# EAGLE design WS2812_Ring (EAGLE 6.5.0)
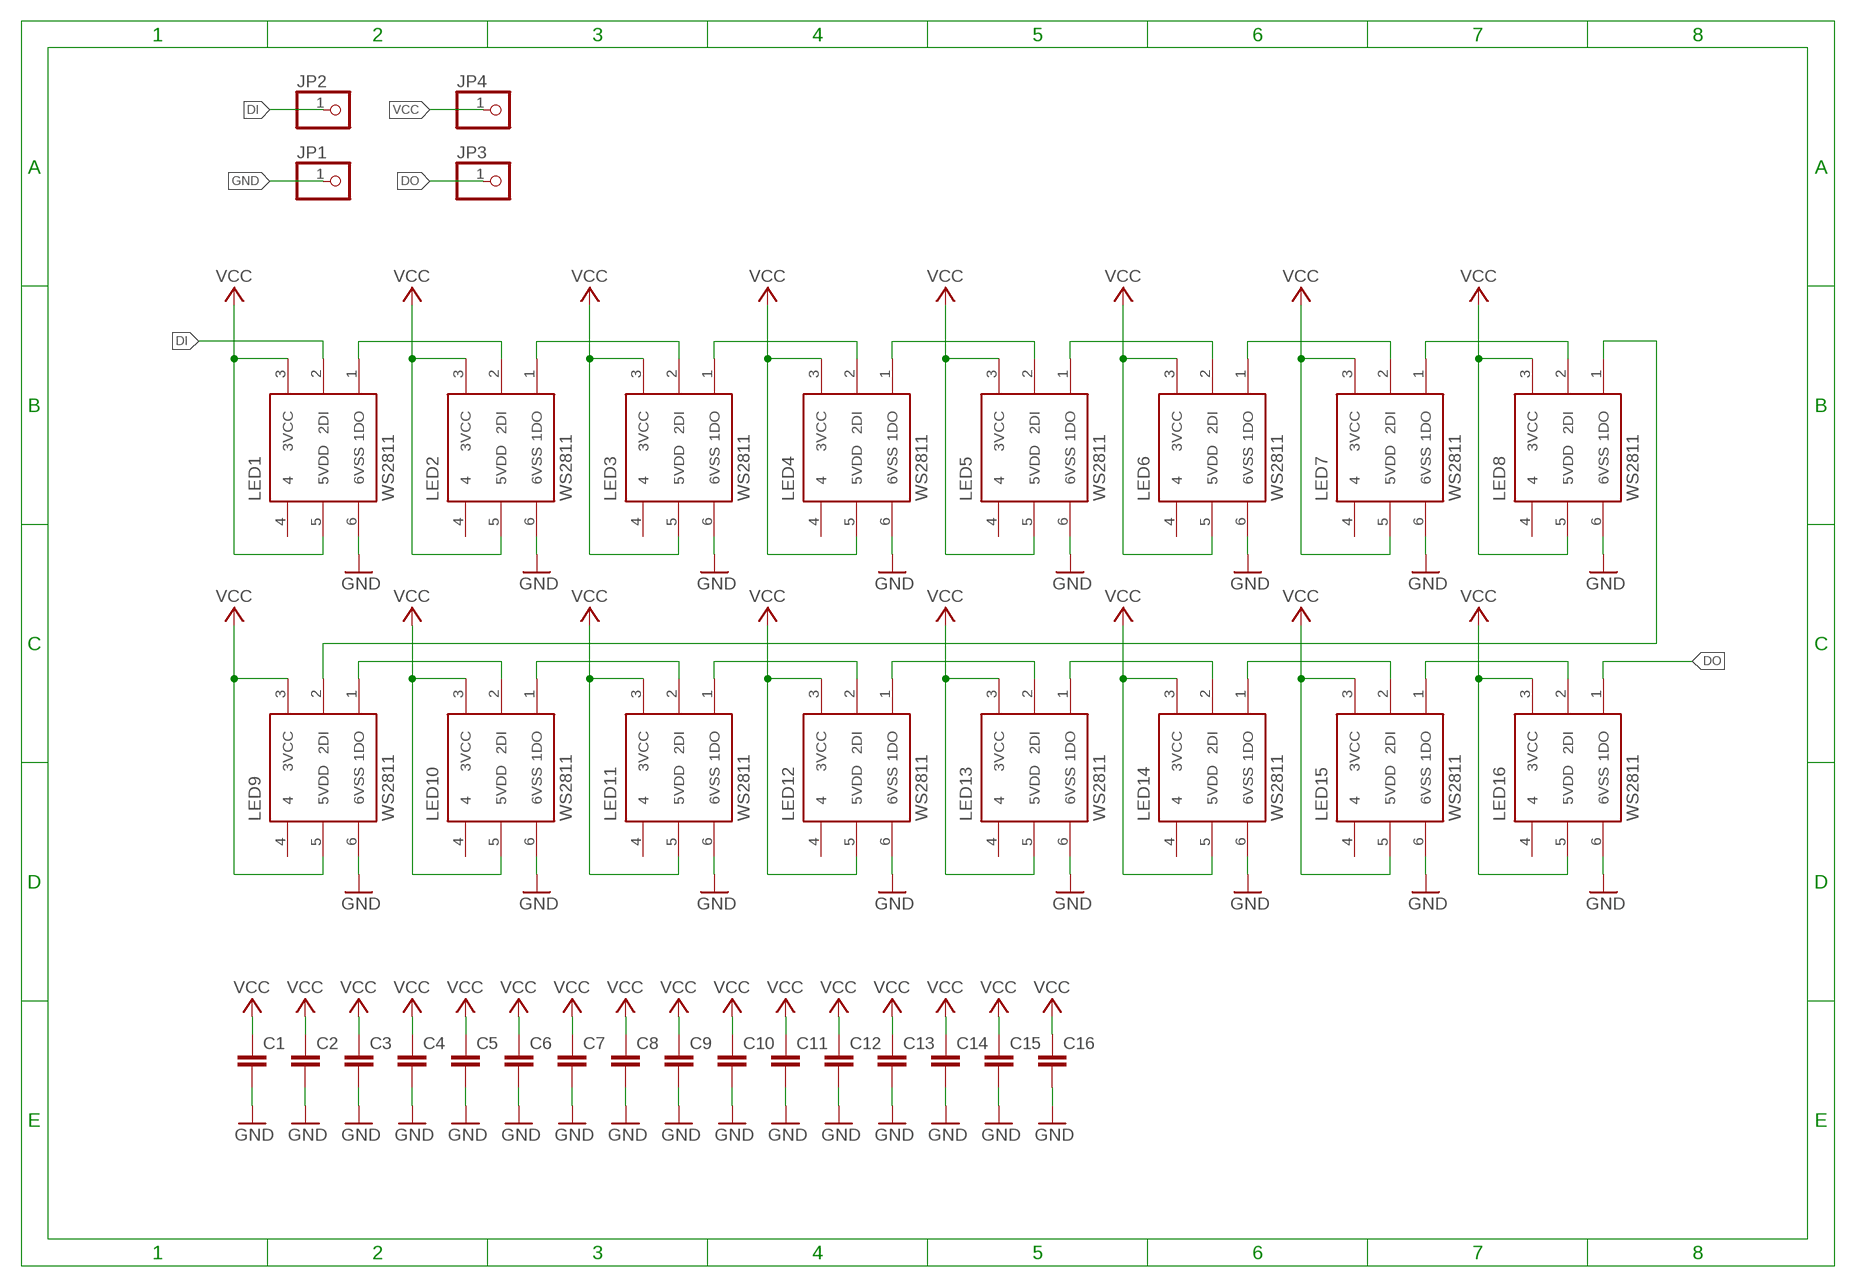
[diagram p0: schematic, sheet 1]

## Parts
C1  C-EUC0805  [C0805]
C2  C-EUC0805  [C0805]
C3  C-EUC0805  [C0805]
C4  C-EUC0805  [C0805]
C5  C-EUC0805  [C0805]
C6  C-EUC0805  [C0805]
C7  C-EUC0805  [C0805]
C8  C-EUC0805  [C0805]
C9  C-EUC0805  [C0805]
C10  C-EUC0805  [C0805]
C11  C-EUC0805  [C0805]
C12  C-EUC0805  [C0805]
C13  C-EUC0805  [C0805]
C14  C-EUC0805  [C0805]
C15  C-EUC0805  [C0805]
C16  C-EUC0805  [C0805]
JP1  PINHD-1X1  [1X01]
JP2  PINHD-1X1  [1X01]
JP3  PINHD-1X1  [1X01]
JP4  PINHD-1X1  [1X01]
LED1  WS2811  [WS2812]
LED2  WS2811  [WS2812]
LED3  WS2811  [WS2812]
LED4  WS2811  [WS2812]
LED5  WS2811  [WS2812]
LED6  WS2811  [WS2812]
LED7  WS2811  [WS2812]
LED8  WS2811  [WS2812]
LED9  WS2811  [WS2812]
LED10  WS2811  [WS2812]
LED11  WS2811  [WS2812]
LED12  WS2811  [WS2812]
LED13  WS2811  [WS2812]
LED14  WS2811  [WS2812]
LED15  WS2811  [WS2812]
LED16  WS2811  [WS2812]

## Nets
DI: JP2.1 LED1.2(2DI)
DO: JP3.1 LED16.1(1DO)
GND: C1.2 C2.2 C3.2 C4.2 C5.2 C6.2 C7.2 C8.2 C9.2 C10.2 C11.2 C12.2 C13.2 C14.2 C15.2 C16.2 JP1.1 LED1.6(6VSS) LED2.6(6VSS) LED3.6(6VSS) LED4.6(6VSS) LED5.6(6VSS) LED6.6(6VSS) LED7.6(6VSS) LED8.6(6VSS) LED9.6(6VSS) LED10.6(6VSS) LED11.6(6VSS) LED12.6(6VSS) LED13.6(6VSS) LED14.6(6VSS) LED15.6(6VSS) LED16.6(6VSS)
N$2: LED1.1(1DO) LED2.2(2DI)
N$3: LED2.1(1DO) LED3.2(2DI)
N$4: LED3.1(1DO) LED4.2(2DI)
N$5: LED4.1(1DO) LED5.2(2DI)
N$6: LED5.1(1DO) LED6.2(2DI)
N$7: LED7.1(1DO) LED8.2(2DI)
N$8: LED9.1(1DO) LED10.2(2DI)
N$9: LED10.1(1DO) LED11.2(2DI)
N$10: LED11.1(1DO) LED12.2(2DI)
N$11: LED12.1(1DO) LED13.2(2DI)
N$12: LED13.1(1DO) LED14.2(2DI)
N$13: LED15.1(1DO) LED16.2(2DI)
N$14: LED8.1(1DO) LED9.2(2DI)
N$15: LED6.1(1DO) LED7.2(2DI)
N$17: LED14.1(1DO) LED15.2(2DI)
VCC: C1.1 C2.1 C3.1 C4.1 C5.1 C6.1 C7.1 C8.1 C9.1 C10.1 C11.1 C12.1 C13.1 C14.1 C15.1 C16.1 JP4.1 LED1.3(3VCC) LED1.5(5VDD) LED2.3(3VCC) LED2.5(5VDD) LED3.3(3VCC) LED3.5(5VDD) LED4.3(3VCC) LED4.5(5VDD) LED5.3(3VCC) LED5.5(5VDD) LED6.3(3VCC) LED6.5(5VDD) LED7.3(3VCC) LED7.5(5VDD) LED8.3(3VCC) LED8.5(5VDD) LED9.3(3VCC) LED9.5(5VDD) LED10.3(3VCC) LED10.5(5VDD) LED11.3(3VCC) LED11.5(5VDD) LED12.3(3VCC) LED12.5(5VDD) LED13.3(3VCC) LED13.5(5VDD) LED14.3(3VCC) LED14.5(5VDD) LED15.3(3VCC) LED15.5(5VDD) LED16.3(3VCC) LED16.5(5VDD)
Unconnected: LED1.4 LED2.4 LED3.4 LED4.4 LED5.4 LED6.4 LED7.4 LED8.4 LED9.4 LED10.4 LED11.4 LED12.4 LED13.4 LED14.4 LED15.4 LED16.4

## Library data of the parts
C1-C16 = rcl:C-EU: CAPACITOR, European symbol
JP1-JP4 = pinhead:PINHD-1X1: PIN HEADER
LED1-LED16 = led2:WS2811

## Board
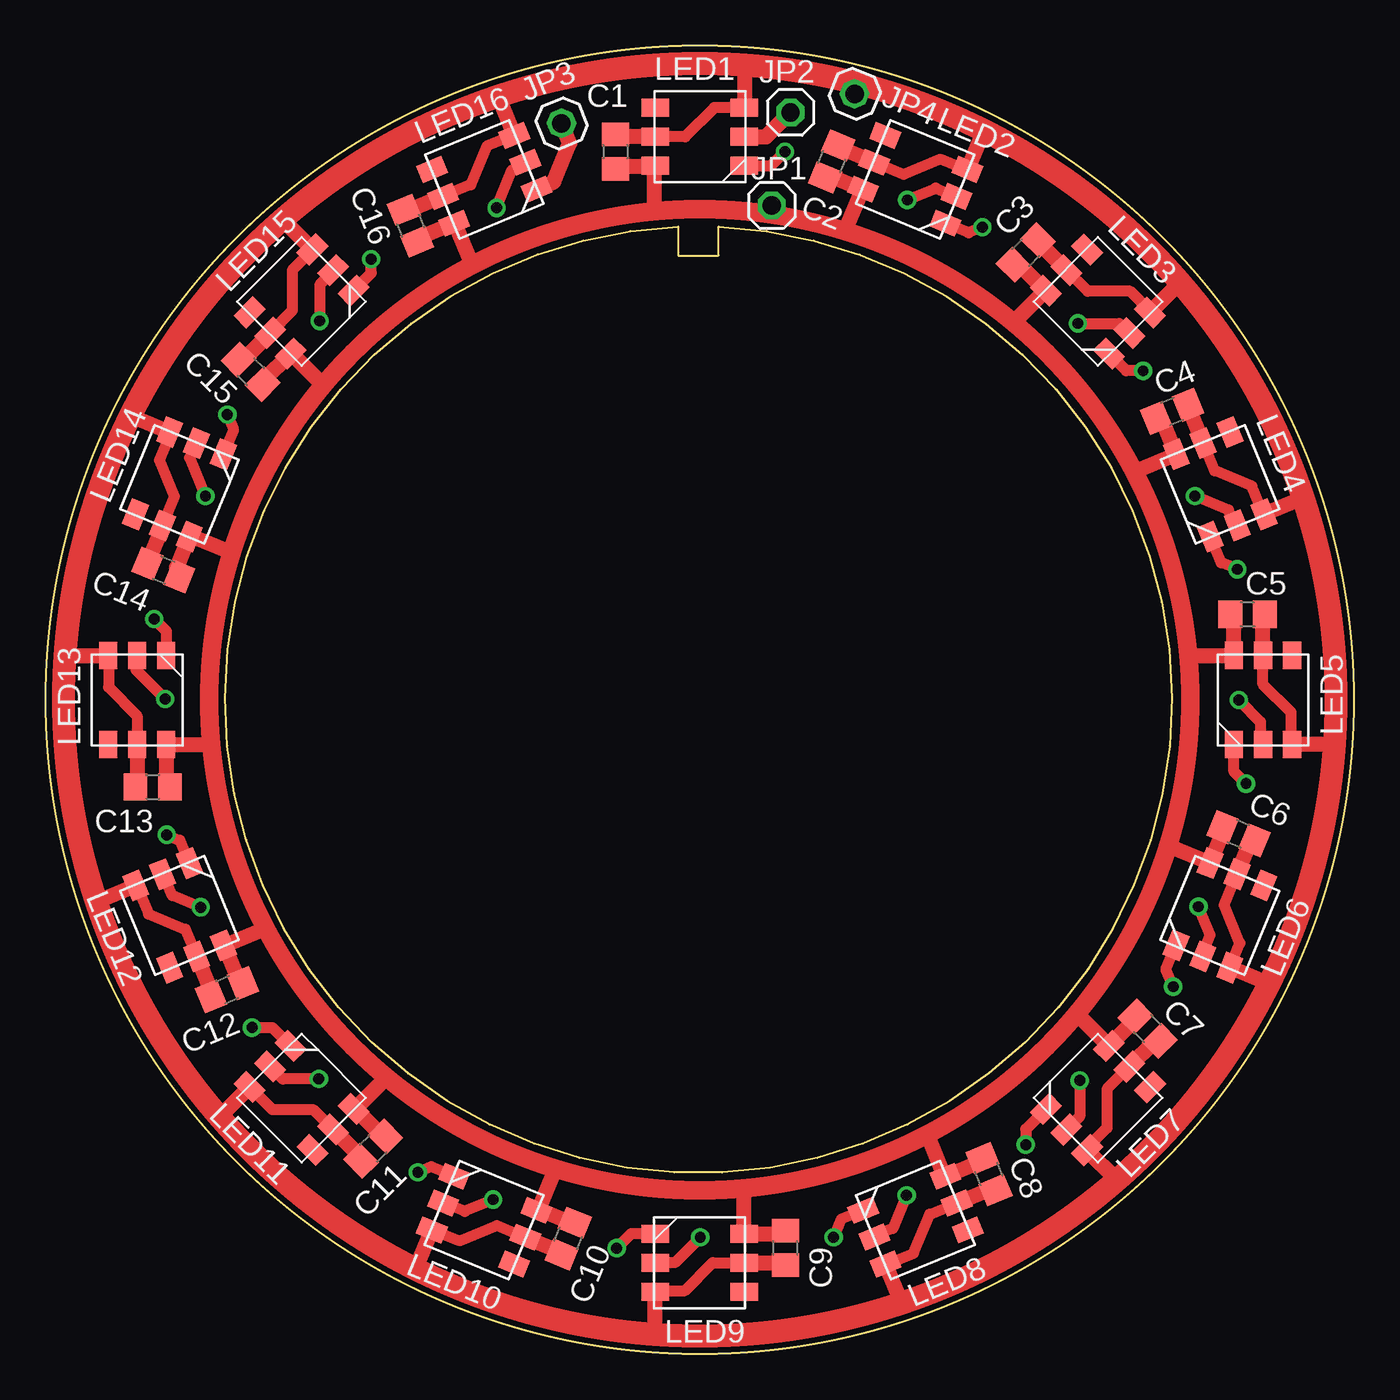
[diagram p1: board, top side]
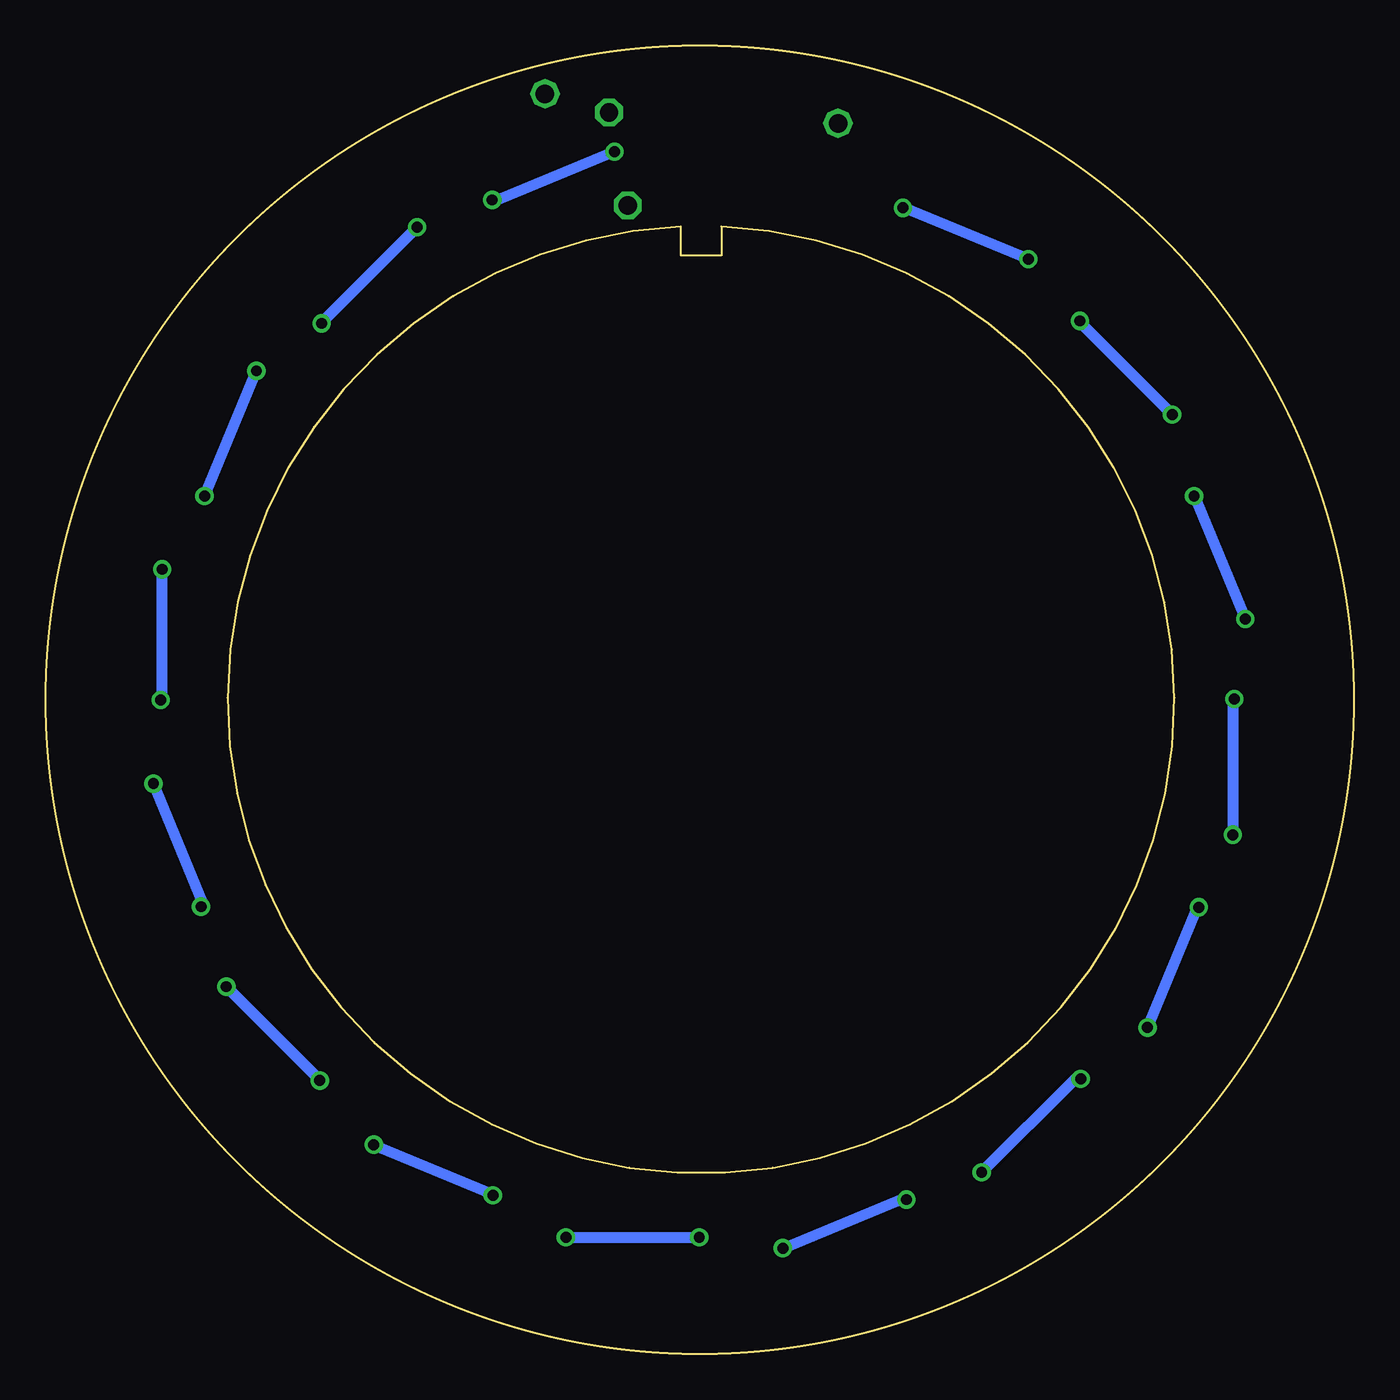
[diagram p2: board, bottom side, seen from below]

Size 72.03 x 72.03 mm. Coordinates in mm from the lower left corner, seen from the top.
Outline: 34.83,62.05 34.83,60.46 37.05,60.46 37.05,62.05 arc-355 34.83,62.05
Outline: circle at 36.01,36.01 radius 36.01
Copper layers (1*16): Top 0.035mm / dielectric 1.5mm / Bottom 0.035mm
Design rules "default": minimum track width 10mil, minimum drill 24mil, track to track 8mil, track to pad 8mil, pad to pad 8mil, via to via 8mil, smd to smd 8mil, copper to edge 40mil, drill to drill 8mil, minimum pad ring 10mil, minimum via ring 8mil, stop-mask expansion 4mil, vias tented up to drill 0mil, thermal gap 10mil

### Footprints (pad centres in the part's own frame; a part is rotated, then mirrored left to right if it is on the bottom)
C0805 = smd 1.3 x 1.5: 1 -0.95,0; 2 0.95,0
1X01 = drill 1.016 octagon: 1 0,0
WS2812 = smd 1.5 x 1: 1 2.45,-1.6; 2 2.45,0; 3 2.45,1.6; 4 -2.45,1.6; 5 -2.45,0; 6 -2.45,-1.6

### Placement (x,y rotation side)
C1  31.37,66.18 270 top
C2  43.28,65.65 247.5 top
C3  53.95,60.63 225 top
C4  62.01,51.88 202.5 top
C5  66.16,40.71 180 top
C6  65.67,28.64 157.5 top
C7  60.66,17.91 135 top
C8  51.93,9.91 112.5 top
C9  40.73,5.85 90 top
C10  28.77,6.35 67.5 top
C11  18.04,11.31 45 top
C12  9.99,20.06 22.5 top
C13  5.9,31.22 0 top
C14  6.49,43.15 337.5 top
C15  11.29,54.07 315 top
C16  20.09,62.1 292.5 top
JP1  39.97,63.22 0 top
JP2  41.01,68.35 0 top
JP3  28.4,67.74 22.5 top
JP4  44.53,69.36 337.5 top
LED1  36.02,67 0 top
LED2  47.88,64.66 337.5 top
LED3  57.93,57.93 315 top
LED4  64.66,47.87 292.5 top
LED5  67.01,36.01 270 top
LED6  64.64,24.15 247.5 top
LED7  57.93,14.09 225 top
LED8  47.89,7.37 202.5 top
LED9  36.01,5.03 180 top
LED10  24.15,7.37 157.5 top
LED11  14.1,14.1 135 top
LED12  7.38,24.14 112.5 top
LED13  5.05,36 90 top
LED14  7.38,47.87 67.5 top
LED15  14.09,57.94 45 top
LED16  24.15,64.66 22.5 top

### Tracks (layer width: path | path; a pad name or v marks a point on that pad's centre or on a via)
DI
  Top 0.813: LED1.2 39.66,67 JP2.1
DO
  Top 0.813: LED16.1 27.98,64.51 28.86,66.63 JP3.1
GND
  Top 0.305: 33.52,65.35 LED1.6 | 61.81,28.01 62.31,30.11 arc17 62.91,34.11 62.91,38.46 62.91,38.51 62.41,41.81 61.41,45.11 60.01,48.61 59.41,49.31 58.01,51.61 55.71,54.51 53.31,56.81 52.61,57.31 51.41,58.11 49.11,59.61 46.61,60.81 44.01,61.81 42.31,62.21 40.01,62.61 37.11,62.91 33.52,62.91 31.02,62.51 | 61.81,28.01 60.81,25.22 59.11,22.02 56.82,18.77 | 56.82,18.77 56.71,18.62 55.01,16.82 52.71,14.82 50.21,13.02 48.51,12.12 45.61,10.72 41.81,9.62 38.41,9.12 34.82,9.02 31.72,9.32 29.32,9.82 28.06,10.18 27.92,10.22 26.02,10.92 23.42,12.02 21.62,13.12 19.72,14.42 18.62,15.32 | 18.62,15.32 17.02,16.82 14.82,19.22 13.52,21.11 12.12,23.51 | 31.02,62.51 28.12,61.81 25.62,60.91 23.52,59.91 | 15.32,53.31 14.92,52.61 13.52,50.91 11.32,46.71 10.22,44.11 9.63,41.85 9.19,39.22 9.04,36.25 9.02,34.1 9.12,33.51 arc7 9.62,30.01 arc15 11.32,25.11 12.12,23.51 | 6.69,33.51 LED13.6 | 61.81,28.01 61.83,27.96 | 56.82,18.67 56.82,18.77 | 49.46,9.82 LED8.6 | 38.41,6.67 LED9.6 | 27.15,7.96 LED10.6 | 17.04,13.5 LED11.6 | 18.62,15.32 18.74,15.2 | 9.84,22.48 LED12.6 | 12.12,23.51 12.15,23.43 | 8,45.03 LED14.6 | 13.56,55.07 LED15.6 | 22.56,62.22 LED16.6 | 44.96,64.1 LED2.6 | 55.03,58.53 LED3.6 | 62.23,49.53 LED4.6 | 65.41,40.51 C5.2 | 64.86,28.85 C6.2 | 59.99,18.41 arc180 C7.2 | 51.49,10.6 arc180 C8.2 | 40.56,6.63 arc180 C9.2 | 29.03,7.18 arc180 C10.2 | 18.55,11.98 C11.2 | 10.65,20.51 C12.2 | 6.65,31.42 C13.2 | 7.21,43.3 7.2,43.29 7.18,43.25 C14.2 | 11.97,53.54 C15.2 | 20.54,61.43 C16.2 | 31.49,65.35 C1.2 | 43.13,64.86 C2.2 | 53.61,59.95 C3.2 | 61.47,51.38 C4.2 | 31.02,62.51 30.67,62.36 JP1.1
  Top 0.813: 33.52,62.91 33.52,65.35 31.49,65.35 | 62.91,38.46 LED5.6 65.41,40.51 | 61.83,27.96 LED6.6 64.86,28.85 | 56.82,18.67 LED7.6 59.99,18.41 | 48.51,12.12 49.46,9.82 | 38.41,9.12 38.41,6.67 | 28.06,10.18 27.15,7.96 29.03,7.18 | 18.74,15.2 17.04,13.5 18.55,11.98 | 12.15,23.43 9.84,22.48 10.65,20.51 | 9.12,33.51 6.69,33.51 | 10.22,44.11 8,45.03 | 15.32,53.31 13.56,55.07 | 23.52,59.91 22.56,62.22 | 44.01,61.81 44.96,64.1 43.13,64.86 | 53.31,56.81 55.03,58.53 53.61,59.95 | 60.01,48.61 62.23,49.53 61.47,51.38 | LED8.6 51.49,10.6 | LED9.6 40.56,6.63 | LED13.6 6.65,31.42 | LED14.6 7.21,43.3 | LED15.6 11.97,53.54 | LED16.6 20.54,61.43
N$2  (via drill 0.6)
  Top 0.305: 50.12,63.71 LED2.2
  Top 0.61: LED1.1 39.93,65.4 v40.71,66.18 | v47.43,63.53 49,64.17 50.12,63.71
  Bottom 0.305: 47.27,63.46 v47.43,63.53
  Bottom 0.61: v40.71,66.18 47.27,63.46
N$3  (via drill 0.6)
  Top 0.305: 59.62,56.2 LED3.2
  Top 0.61: LED2.1 50.81,61.71 v51.58,62.03 | v56.83,56.73 59.09,56.73 59.62,56.2
  Bottom 0.305: 56.83,56.77 v56.83,56.73
  Bottom 0.61: v51.58,62.03 56.83,56.77
N$4  (via drill 0.6)
  Top 0.305: LED4.2 65.44,45.67 | 65.12,46.46 65.54,45.43 65.56,45.42
  Top 0.61: 65.44,45.67 65.12,46.46 v63.27,47.22 | LED3.1 59.48,54.12 v60.41,54.12
  Bottom 0.61: v63.27,47.22 v60.41,54.12
N$5  (via drill 0.6)
  Top 0.305: 66.88,33.69 LED5.2
  Top 0.61: LED4.1 64.71,43.56 v65.6,43.2 | v65.68,36 66.88,34.8 66.88,33.69
  Bottom 0.305: v65.68,36 65.6,36.07
  Bottom 0.61: 65.6,36.07 v65.6,43.2
N$6  (via drill 0.6)
  Top 0.305: LED6.2 63.67,21.98
  Top 0.61: LED5.1 65.41,32.06 v66.08,31.4 | v63.46,24.62 64.11,23.06 63.67,21.98
  Bottom 0.305: v63.46,24.62 63.37,24.85
  Bottom 0.61: 63.37,24.85 v66.08,31.4
N$7  (via drill 0.6)
  Top 0.305: 45.65,6.5 LED8.2
  Top 0.61: LED7.1 53.96,12.38 v53.96,11.52 | v47.4,8.74 46.64,6.91 45.65,6.5
  Bottom 0.305: 47.43,8.82 v47.4,8.74
  Bottom 0.61: v53.96,11.52 47.43,8.82
N$8  (via drill 0.6)
  Top 0.305: 21.93,8.33 LED10.2
  Top 0.61: LED9.1 32.24,6.63 v31.44,5.83 | v24.64,8.5 23.07,7.85 21.93,8.33
  Bottom 0.305: 24.81,8.58 v24.64,8.5
  Bottom 0.61: v31.44,5.83 24.81,8.58
N$9  (via drill 0.6)
  Top 0.305: 12.39,15.83 LED11.2
  Top 0.61: LED10.1 21.24,10.31 v20.5,10 | v15.05,15.15 13.07,15.15 12.39,15.83
  Bottom 0.305: 15.35,15.15 v15.05,15.15
  Bottom 0.61: v20.5,10 15.35,15.15
N$10  (via drill 0.6)
  Top 0.305: 6.51,26.38 LED12.2
  Top 0.61: LED11.1 12.48,17.97 v11.37,17.97 | v8.55,24.59 6.98,25.24 6.51,26.38
  Bottom 0.305: v8.55,24.59 8.65,24.55
  Bottom 0.61: 8.65,24.55 v11.37,17.97
N$11  (via drill 0.6)
  Top 0.305: 4.99,37.65 4.99,38.38 LED13.2
  Top 0.61: LED12.1 7.4,28.28 v6.68,28.58 | 4.99,37.65 v6.59,36.05
  Bottom 0.305: v6.59,36.05 6.68,35.96
  Bottom 0.61: 6.68,35.96 v6.68,28.58
N$12  (via drill 0.6)
  Top 0.305: LED14.2 8.27,50.12
  Top 0.61: LED13.1 6.65,39.79 v5.99,40.45 | v8.81,47.23 7.94,49.32 8.27,50.12
  Bottom 0.305: v8.81,47.23 8.79,47.22
  Bottom 0.61: 8.79,47.22 v5.99,40.45
N$13  (via drill 0.6)
  Top 0.305: 26.36,65.46 LED16.2
  Top 0.61: LED15.1 17.93,59.5 v17.93,60.26 | v24.83,63.09 25.69,65.18 26.36,65.46
  Bottom 0.305: 24.79,63.11 v24.83,63.09
  Bottom 0.61: v17.93,60.26 24.79,63.11
N$14  (via drill 0.6)
  Top 0.305: LED9.2
  Top 0.61: LED8.1 43.79,7.41 v43.38,6.42 | v36.04,6.43 34.64,5.03 LED9.2
  Bottom 0.305: v36.05,6.42 v36.04,6.43
  Bottom 0.61: v43.38,6.42 v36.05,6.42
N$15  (via drill 0.6)
  Top 0.305: LED7.2
  Top 0.61: LED6.1 61.68,21.17 v62.07,20.22 | v56.93,15.06 56.93,13.08 LED7.2
  Bottom 0.305: v56.93,15.06 56.93,15.08
  Bottom 0.61: 56.93,15.08 v62.07,20.22
N$17  (via drill 0.6)
  Top 0.305: LED15.2 15.83,59.58
  Top 0.61: LED14.1 10.35,50.88 v10.01,51.71 | v15.1,56.87 15.1,58.85 15.83,59.58
  Bottom 0.305: v15.1,56.87 15.1,56.79
  Bottom 0.61: 15.1,56.79 v10.01,51.71
VCC
  Top 0.305: 38.47,70.46 39.01,71.01 40.01,71.01 41.11,70.65 44.74,70.01 48.14,68.82 51.65,67.36 | LED1.3 | LED6.3 | 57.33,11.34 LED7.3 | 58.95,9.61 59,9.61 | 59,9.61 62.67,13.29 64.51,15.69 66.35,18.66 67.35,20.37 67.43,20.4 67.41,20.37 arc179 67.43,20.33 68.88,23.84 69.69,26.32 70.52,29.88 70.81,33.56 70.96,33.71 70.96,36.71 70.76,39.91 70.36,42.71 69.56,45.51 69,47.02 69.16,47.4 67.85,50.54 66.29,53.79 64.33,56.44 62.39,58.92 | LED8.3 46.28,4.94 | 59,9.61 56.45,7.63 53.72,5.85 50.37,4.03 47.22,2.73 47.15,2.76 42.79,1.69 39.99,1.29 37.39,1.09 33.59,1.09 33.56,1.12 30.95,1.35 27.58,2.09 24.11,3.1 20.41,4.63 20.39,4.69 17.29,6.39 14.32,8.52 11.78,10.78 9.87,12.68 | LED9.3 33.63,3.49 | LED10.3 21.32,6.85 | LED11.3 11.25,14.7 | 9.65,13.12 9.65,12.9 9.87,12.68 | LED12.3 5.04,25.76 | 2.77,24.96 2.86,24.92 | 2.77,24.96 4.38,21.08 6.92,16.51 9.87,12.68 | LED13.3 3.47,38.43 | 1.07,38.5 1.13,38.45 | 1.07,38.5 1.07,33.3 1.47,30.5 2.27,26.7 2.77,24.96 | LED14.3 6.88,50.64 | 4.67,51.59 4.74,51.62 | 4.67,51.59 3.45,48.63 2.33,45.42 1.31,40.86 1.07,38.5 | LED15.3 14.7,60.75 | 13.03,62.47 13.02,62.47 | 13.03,62.47 10.34,59.79 7.93,57.1 4.67,51.59 | LED16.3 25.77,67.09 | 24.96,69.11 24.93,69.12 21.71,68 17.8,65.95 15.07,64.17 13.03,62.47 | LED2.3 50.68,65.17 | 51.65,67.36 | LED3.3 60.8,57.41 | 62.39,58.92 | 62.39,58.92 60.84,60.76 56.74,64.29 51.65,67.36 | LED4.3 67.04,46.24 | LED5.3 68.56,33.61 | 67.01,40.62 arc-53 C5.1 | 66.31,28.17 arc-180 C6.1 | 61.08,17.23 arc-180 C7.1 | 52.09,9.12 arc-180 C8.1 | 40.59,5.03 arc-180 C9.1 | 28.34,5.63 arc-53 C10.1 | 17.37,10.83 C11.1 | 9.17,19.83 C12.1 | 5.05,31.31 C13.1 | LED14.5 6.46,45.56
  Top 0.305: 10.9,54.74 C15.1 | 19.92,62.9 C16.1 | 31.5,67 C1.1 | 43.7,66.39 C2.1 | 54.63,61.24 C3.1 | 62.87,52.2 C4.1
  Top 0.61: LED1.5 35.21,67 36.81,68.61 LED1.3 | LED6.5 64.88,24.71 65.75,22.62 LED6.3 | LED7.5 58.43,14.59 58.43,12.44 57.33,11.34 | LED8.5 48.67,7.7 47.78,5.56 46.28,4.94 | LED9.5 36.72,5.03 35.19,3.49 33.63,3.49 | LED10.5 24.85,7.08 22.81,6.24 21.32,6.85 | LED11.5 14.73,13.47 12.48,13.46 11.25,14.7 | LED12.5 7.7,23.38 5.68,24.22 5.04,25.76 | LED13.5 5.05,35.12 3.47,36.7 3.47,38.43 | LED14.5 7.1,47.2 6.28,49.19 6.88,50.64 | LED15.5 13.59,57.43 13.59,59.65 14.7,60.75 | LED16.5 23.41,64.35 24.29,66.48 25.77,67.09 | LED2.5 47.24,64.92 49.26,65.76 50.68,65.17 | LED3.5 57.37,58.5 59.71,58.5 60.8,57.41 | LED4.5 64.35,48.62 66.4,47.77 67.04,46.24 | LED5.5 67.01,36.86 68.56,35.31 68.56,33.61
  Top 0.813: 38.47,70.46 LED1.3 | 67.35,20.37 LED6.3 | LED7.3 58.95,9.61 | 47.15,2.76 LED8.3 | 33.56,1.12 LED9.3 | 20.39,4.69 LED10.3 | 9.65,13.12 LED11.3 | 2.86,24.92 LED12.3 | 1.13,38.45 LED13.3 | 4.74,51.62 LED14.3 | 13.02,62.47 LED15.3 | 24.96,69.11 LED16.3 | 51.65,67.36 LED2.3 | 62.39,58.92 LED3.3 | 69,47.02 LED4.3 | 70.81,33.56 LED5.3 | LED5.5 67.01,40.62 | LED6.5 66.31,28.17 | LED7.5 61.08,17.23 | LED8.5 52.09,9.12 | LED9.5 40.59,5.03 | LED10.5 28.34,5.63 | LED11.5 17.37,10.83 | LED12.5 9.17,19.83 | LED13.5 5.05,31.31 | 6.46,45.56 C14.1 | LED15.5 10.9,54.74 | LED16.5 19.92,62.9 | LED1.5 31.5,67 | LED2.5 43.7,66.39 | LED3.5 54.63,61.24 | LED4.5 62.87,52.2 | 44.74,70.01 44.5,69.44 JP4.1
(copper drawn outside any net)
  shapes: Top circle x2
